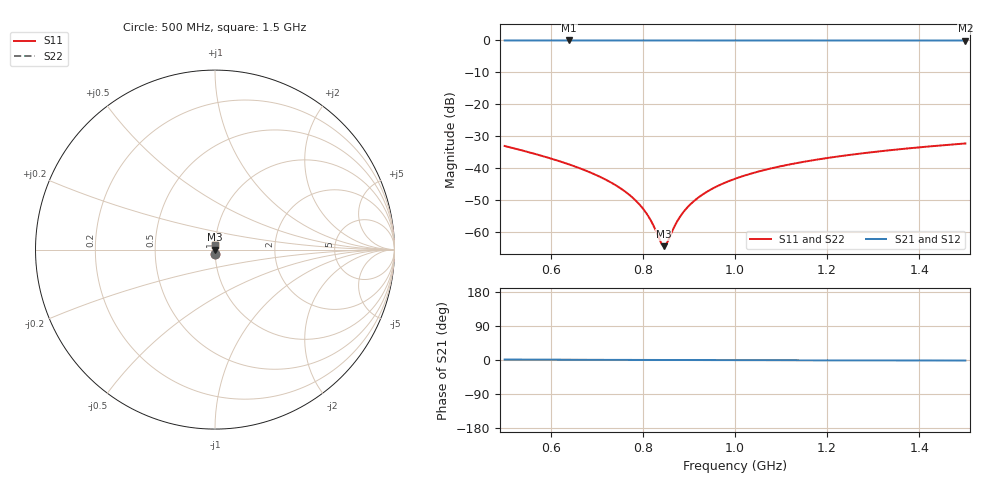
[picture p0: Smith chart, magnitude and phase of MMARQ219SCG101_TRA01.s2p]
! MMARQ219SCG101_TRA01  S-PARAMETER MODEL  ( General Type )
! Model Generated by TAIYO YUDEN Corporation (http://www.ty-top.com)
! Version 1.0
! TAIYO YUDEN Control No. 150609
! Copyright(c) 2015 TAIYO YUDEN CO.,LTD. All Rights Reserved.
! Product Description (link to TY-COMPAS)
! https://ds.yuden.co.jp/TYCOMPAS/or/detail?pn=MMARQ219SCG101JTRA01&u=M
! Products Name : Multilayer Ceramic Capacitors
! Characteristics :
!  Capacitance : 100 pF , Rated Voltage : 250V , TCC : CG / C0G
!  Case Size : 2.0 x 1.25 / 0.079 x 0.049 [mm/inch] , Thickness : 0.85 / 0.033 [mm/inch]
!  (Conditions: Temperature = 25 degC , DC Bias Current/Voltage = 0A / 0V)
! External Node Assignments :
!  1  o---| |---o  2
! GND o---------o GND
! Frequency Range : 500MHz  -  1.5GHz  [ 401 STEP ]
# MHz S RI R 50
! Freq[MHz].  S11 Real  S11 Imag  S21 Real  S21 Imag  S12 Real  S12 Imag  S22 Real  S22 Imag
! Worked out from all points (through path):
!   401 points, 500 MHz to 1.5 GHz, reference 50 ohm
!   highest |S21| = 0.00 dB at 640 MHz (marker M1); lowest = 0.0 dB at 1.5 GHz (marker M2)
!   lowest |S11| = -64.4 dB at 845 MHz (marker M3), VSWR 1.00, Z = 50.1 - j0.00634 ohm
!   |S11| at or under -10 dB: start of sweep to end of sweep
!   |S22| runs from -64.4 to -32.3 dB; largest |S21 - S12| = 0
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500  0.000806 -0.0222  0.9992 0.0222  0.9992 0.0222  0.000806 -0.0222
640  0.0005 -0.0114  0.9995 0.0114  0.9995 0.0114  0.0005 -0.0114
667.5  0.000485 -0.00967  0.9995 0.00967  0.9995 0.00967  0.000485 -0.00967
730  0.000488 -0.00599  0.9995 0.00599  0.9995 0.00599  0.000488 -0.00599
755  0.000502 -0.00462  0.9995 0.00462  0.9995 0.00462  0.000502 -0.00462
777.5  0.000519 -0.00343  0.9995 0.00343  0.9995 0.00343  0.000519 -0.00343
795  0.000535 -0.00253  0.9995 0.00253  0.9995 0.00253  0.000535 -0.00253
810  0.000552 -0.00177  0.9994 0.00177  0.9994 0.00177  0.000552 -0.00177
822.5  0.000566 -0.00115  0.9994 0.00115  0.9994 0.00115  0.000566 -0.00115
835  0.000582 -0.000543  0.9994 0.000543  0.9994 0.000543  0.000582 -0.000543
840  0.000589 -0.000303  0.9994 0.000303  0.9994 0.000303  0.000589 -0.000303
845  0.000596 -6.33e-05  0.9994 6.33e-05  0.9994 6.33e-05  0.000596 -6.33e-05
852.5  0.000607 0.000293  0.9994 -0.000293  0.9994 -0.000293  0.000607 0.000293
870  0.000633 0.00111  0.9994 -0.00111  0.9994 -0.00111  0.000633 0.00111
880  0.000649 0.00157  0.9994 -0.00157  0.9994 -0.00157  0.000649 0.00157
905  0.000692 0.0027  0.9993 -0.0027  0.9993 -0.0027  0.000692 0.0027
945  0.000769 0.00445  0.9992 -0.00445  0.9992 -0.00445  0.000769 0.00445
1000  0.000889 0.00675  0.9991 -0.00675  0.9991 -0.00675  0.000889 0.00675
1072.5  0.00107 0.00962  0.9989 -0.00962  0.9989 -0.00962  0.00107 0.00962
1167.5  0.00135 0.0132  0.9987 -0.0132  0.9987 -0.0132  0.00135 0.0132
1335  0.00192 0.0189  0.9981 -0.0189  0.9981 -0.0189  0.00192 0.0189
1500  0.00258 0.0242  0.9974 -0.0242  0.9974 -0.0242  0.00258 0.0242
